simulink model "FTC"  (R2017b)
settings: Solver=FixedStepDiscrete  StartTime=0.0  StopTime=10.0  FixedStep=0.01  RelTol=1e-3  EnableMultiTasking=on
undefined symbols (not defined in the file): ASWTYPE_TRUE, Enum_CMSHVBatFltSevrtyStat
libraries: AIWAYS_Powertrain_BMS_lib x22

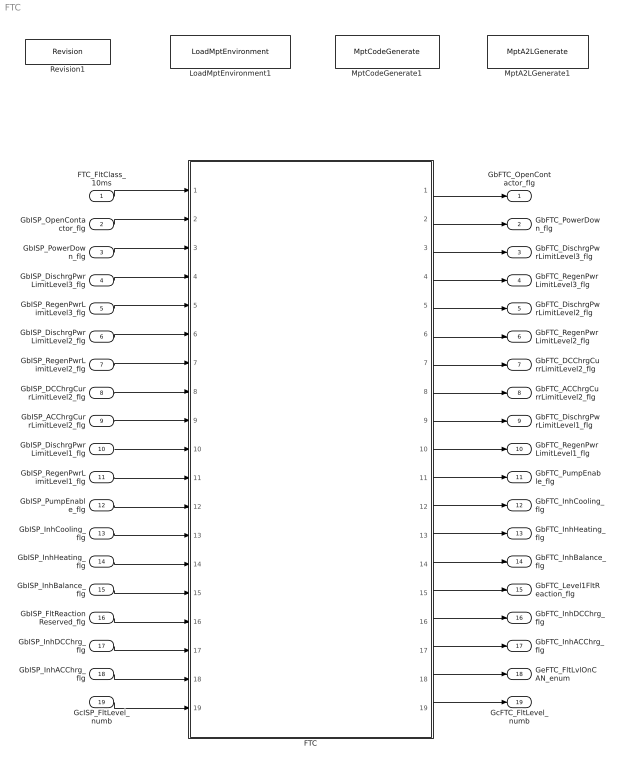
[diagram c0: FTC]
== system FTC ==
  FTC_FltClass_10ms : Inport
  GbISP_OpenContactor_flg : Inport  Port=2
  GbISP_PowerDown_flg : Inport  Port=3
  GbISP_DischrgPwrLimitLevel3_flg : Inport  Port=4
  GbISP_RegenPwrLimitLevel3_flg : Inport  Port=5
  GbISP_DischrgPwrLimitLevel2_flg : Inport  Port=6
  GbISP_RegenPwrLimitLevel2_flg : Inport  Port=7
  GbISP_DCChrgCurrLimitLevel2_flg : Inport  Port=8
  GbISP_ACChrgCurrLimitLevel2_flg : Inport  Port=9
  GbISP_DischrgPwrLimitLevel1_flg : Inport  Port=10
  GbISP_RegenPwrLimitLevel1_flg : Inport  Port=11
  GbISP_PumpEnable_flg : Inport  Port=12
  GbISP_InhCooling_flg : Inport  Port=13
  GbISP_InhHeating_flg : Inport  Port=14
  GbISP_InhBalance_flg : Inport  Port=15
  GbISP_FltReactionReserved_flg : Inport  Port=16
  GbISP_InhDCChrg_flg : Inport  Port=17
  GbISP_InhACChrg_flg : Inport  Port=18
  GcISP_FltLevel_numb : Inport  Port=19
  FTC : Subsystem
  LoadMptEnvironment1 : AIWAYS_Powertrain_BMS_lib/Config/LoadMptEnvironment  ProjectName=Comm  SuppierID=NewPlatformUAES
  MptA2LGenerate1 : AIWAYS_Powertrain_BMS_lib/Config/MptA2LGenerate  SystemSampleTime=-1
  MptCodeGenerate1 : AIWAYS_Powertrain_BMS_lib/Config/MptCodeGenerate  SystemSampleTime=-1
  Revision1 : AIWAYS_Powertrain_BMS_lib/Config/Revision  curVersion='M103C105'  newVersion='M103C105'
  GbFTC_OpenContactor_flg : Outport
  GbFTC_PowerDown_flg : Outport  Port=2
  GbFTC_DischrgPwrLimitLevel3_flg : Outport  Port=3
  GbFTC_RegenPwrLimitLevel3_flg : Outport  Port=4
  GbFTC_DischrgPwrLimitLevel2_flg : Outport  Port=5
  GbFTC_RegenPwrLimitLevel2_flg : Outport  Port=6
  GbFTC_DCChrgCurrLimitLevel2_flg : Outport  Port=7
  GbFTC_ACChrgCurrLimitLevel2_flg : Outport  Port=8
  GbFTC_DischrgPwrLimitLevel1_flg : Outport  Port=9
  GbFTC_RegenPwrLimitLevel1_flg : Outport  Port=10
  GbFTC_PumpEnable_flg : Outport  Port=11
  GbFTC_InhCooling_flg : Outport  Port=12
  GbFTC_InhHeating_flg : Outport  Port=13
  GbFTC_InhBalance_flg : Outport  Port=14
  GbFTC_Level1FltReaction_flg : Outport  Port=15
  GbFTC_InhDCChrg_flg : Outport  Port=16
  GbFTC_InhACChrg_flg : Outport  Port=17
  GeFTC_FltLvlOnCAN_enum : Outport  Port=18
  GcFTC_FltLevel_numb : Outport  Port=19
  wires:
  FTC_FltClass_10ms/1 -> FTC/1(FTC_FltClass_10ms)
  GbISP_OpenContactor_flg/1 -> FTC/2(GbISP_OpenContactor_flg)
  GbISP_PowerDown_flg/1 -> FTC/3(GbISP_PowerDown_flg)
  GbISP_DischrgPwrLimitLevel3_flg/1 -> FTC/4(GbISP_DischrgPwrLimitLevel3_flg)
  GbISP_RegenPwrLimitLevel3_flg/1 -> FTC/5(GbISP_RegenPwrLimitLevel3_flg)
  GbISP_DischrgPwrLimitLevel2_flg/1 -> FTC/6(GbISP_DischrgPwrLimitLevel2_flg)
  GbISP_RegenPwrLimitLevel2_flg/1 -> FTC/7(GbISP_RegenPwrLimitLevel2_flg)
  GbISP_DCChrgCurrLimitLevel2_flg/1 -> FTC/8(GbISP_DCChrgCurrLimitLevel2_flg)
  GbISP_ACChrgCurrLimitLevel2_flg/1 -> FTC/9(GbISP_ACChrgCurrLimitLevel2_flg)
  GbISP_DischrgPwrLimitLevel1_flg/1 -> FTC/10(GbISP_DischrgPwrLimitLevel1_flg)
  GbISP_RegenPwrLimitLevel1_flg/1 -> FTC/11(GbISP_RegenPwrLimitLevel1_flg)
  GbISP_PumpEnable_flg/1 -> FTC/12(GbISP_PumpEnable_flg)
  GbISP_InhCooling_flg/1 -> FTC/13(GbISP_InhCooling_flg)
  GbISP_InhHeating_flg/1 -> FTC/14(GbISP_InhHeating_flg)
  GbISP_InhBalance_flg/1 -> FTC/15(GbISP_InhBalance_flg)
  GbISP_FltReactionReserved_flg/1 -> FTC/16(GbISP_Level1FltReaction_flg)
  FTC/1(GbFTC_OpenContactor_flg) -> GbFTC_OpenContactor_flg/1
  FTC/2(GbFTC_PowerDown_flg) -> GbFTC_PowerDown_flg/1
  FTC/3(GbFTC_DischrgPwrLimitLevel3_flg) -> GbFTC_DischrgPwrLimitLevel3_flg/1
  FTC/4(GbFTC_RegenPwrLimitLevel3_flg) -> GbFTC_RegenPwrLimitLevel3_flg/1
  FTC/5(GbFTC_DischrgPwrLimitLevel2_flg) -> GbFTC_DischrgPwrLimitLevel2_flg/1
  FTC/6(GbFTC_RegenPwrLimitLevel2_flg) -> GbFTC_RegenPwrLimitLevel2_flg/1
  FTC/7(GbFTC_DCChrgCurrLimitLevel2_flg) -> GbFTC_DCChrgCurrLimitLevel2_flg/1
  FTC/8(GbFTC_ACChrgCurrLimitLevel2_flg) -> GbFTC_ACChrgCurrLimitLevel2_flg/1
  FTC/9(GbFTC_DischrgPwrLimitLevel1_flg) -> GbFTC_DischrgPwrLimitLevel1_flg/1
  FTC/10(GbFTC_RegenPwrLimitLevel1_flg) -> GbFTC_RegenPwrLimitLevel1_flg/1
  FTC/11(GbFTC_PumpEnable_flg) -> GbFTC_PumpEnable_flg/1
  FTC/12(GbFTC_InhCooling_flg) -> GbFTC_InhCooling_flg/1
  FTC/13(GbFTC_InhHeating_flg) -> GbFTC_InhHeating_flg/1
  FTC/14(GbFTC_InhBalance_flg) -> GbFTC_InhBalance_flg/1
  FTC/15(GbFTC_Level1FltReaction_flg) -> GbFTC_Level1FltReaction_flg/1
  FTC/16(GbFTC_InhDCChrg_flg) -> GbFTC_InhDCChrg_flg/1
  FTC/17(GbFTC_InhACChrg_flg) -> GbFTC_InhACChrg_flg/1
  GbISP_InhDCChrg_flg/1 -> FTC/17(GbISP_InhDCChrg_flg)
  GbISP_InhACChrg_flg/1 -> FTC/18(GbISP_InhACChrg_flg)
  FTC/18(GeFTC_FltLvlOnCAN_enum) -> GeFTC_FltLvlOnCAN_enum/1
  GcISP_FltLevel_numb/1 -> FTC/19(GcISP_FltLevel_numb)
  FTC/19(GcFTC_FltLevel_numb) -> GcFTC_FltLevel_numb/1

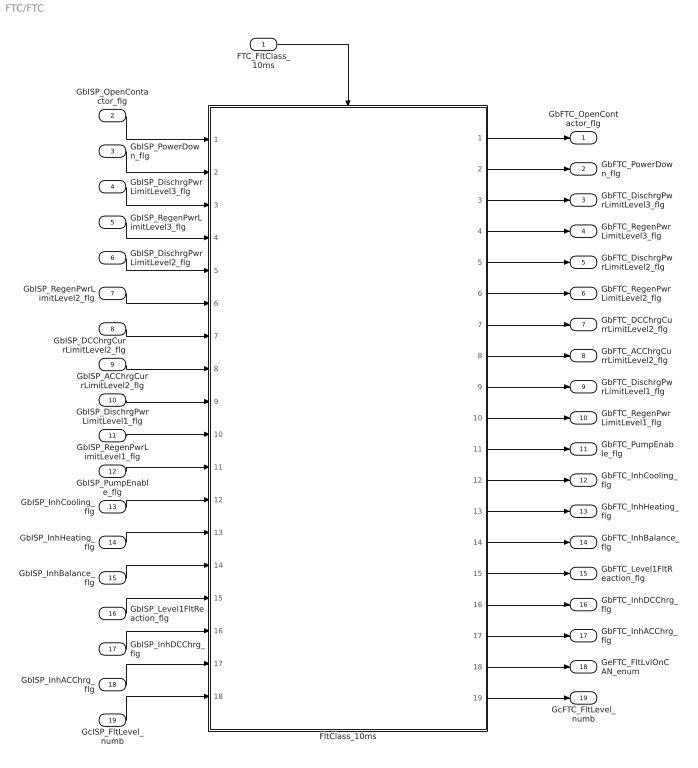
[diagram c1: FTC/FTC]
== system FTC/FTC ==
  FTC_FltClass_10ms : Inport
  GbISP_OpenContactor_flg : Inport  Port=2
  GbISP_PowerDown_flg : Inport  Port=3
  GbISP_DischrgPwrLimitLevel3_flg : Inport  Port=4
  GbISP_RegenPwrLimitLevel3_flg : Inport  Port=5
  GbISP_DischrgPwrLimitLevel2_flg : Inport  Port=6
  GbISP_RegenPwrLimitLevel2_flg : Inport  Port=7
  GbISP_DCChrgCurrLimitLevel2_flg : Inport  Port=8
  GbISP_ACChrgCurrLimitLevel2_flg : Inport  Port=9
  GbISP_DischrgPwrLimitLevel1_flg : Inport  Port=10
  GbISP_RegenPwrLimitLevel1_flg : Inport  Port=11
  GbISP_PumpEnable_flg : Inport  Port=12
  GbISP_InhCooling_flg : Inport  Port=13
  GbISP_InhHeating_flg : Inport  Port=14
  GbISP_InhBalance_flg : Inport  Port=15
  GbISP_Level1FltReaction_flg : Inport  Port=16
  GbISP_InhDCChrg_flg : Inport  Port=17
  GbISP_InhACChrg_flg : Inport  Port=18
  GcISP_FltLevel_numb : Inport  Port=19
  FltClass_10ms : Subsystem
  GbFTC_OpenContactor_flg : Outport
  GbFTC_PowerDown_flg : Outport  Port=2
  GbFTC_DischrgPwrLimitLevel3_flg : Outport  Port=3
  GbFTC_RegenPwrLimitLevel3_flg : Outport  Port=4
  GbFTC_DischrgPwrLimitLevel2_flg : Outport  Port=5
  GbFTC_RegenPwrLimitLevel2_flg : Outport  Port=6
  GbFTC_DCChrgCurrLimitLevel2_flg : Outport  Port=7
  GbFTC_ACChrgCurrLimitLevel2_flg : Outport  Port=8
  GbFTC_DischrgPwrLimitLevel1_flg : Outport  Port=9
  GbFTC_RegenPwrLimitLevel1_flg : Outport  Port=10
  GbFTC_PumpEnable_flg : Outport  Port=11
  GbFTC_InhCooling_flg : Outport  Port=12
  GbFTC_InhHeating_flg : Outport  Port=13
  GbFTC_InhBalance_flg : Outport  Port=14
  GbFTC_Level1FltReaction_flg : Outport  Port=15
  GbFTC_InhDCChrg_flg : Outport  Port=16
  GbFTC_InhACChrg_flg : Outport  Port=17
  GeFTC_FltLvlOnCAN_enum : Outport  Port=18
  GcFTC_FltLevel_numb : Outport  Port=19
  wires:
  GbISP_OpenContactor_flg/1 -> FltClass_10ms/1(GbISP_OpenContactor_flg)
  GbISP_PowerDown_flg/1 -> FltClass_10ms/2(GbISP_PowerDown_flg)
  GbISP_DischrgPwrLimitLevel3_flg/1 -> FltClass_10ms/3(GbISP_DischrgPwrLimitLevel3_flg)
  GbISP_RegenPwrLimitLevel3_flg/1 -> FltClass_10ms/4(GbISP_RegenPwrLimitLevel3_flg)
  GbISP_DischrgPwrLimitLevel2_flg/1 -> FltClass_10ms/5(GbISP_DischrgPwrLimitLevel2_flg)
  GbISP_RegenPwrLimitLevel2_flg/1 -> FltClass_10ms/6(GbISP_RegenPwrLimitLevel2_flg)
  GbISP_DCChrgCurrLimitLevel2_flg/1 -> FltClass_10ms/7(GbISP_DCChrgCurrLimitLevel2_flg)
  GbISP_ACChrgCurrLimitLevel2_flg/1 -> FltClass_10ms/8(GbISP_ACChrgCurrLimitLevel2_flg)
  GbISP_DischrgPwrLimitLevel1_flg/1 -> FltClass_10ms/9(GbISP_DischrgPwrLimitLevel1_flg)
  GbISP_RegenPwrLimitLevel1_flg/1 -> FltClass_10ms/10(GbISP_RegenPwrLimitLevel1_flg)
  GbISP_PumpEnable_flg/1 -> FltClass_10ms/11(GbISP_PumpEnable_flg)
  GbISP_InhCooling_flg/1 -> FltClass_10ms/12(GbISP_InhCooling_flg)
  GbISP_InhHeating_flg/1 -> FltClass_10ms/13(GbISP_InhHeating_flg)
  GbISP_InhBalance_flg/1 -> FltClass_10ms/14(GbISP_InhBalance_flg)
  GbISP_Level1FltReaction_flg/1 -> FltClass_10ms/15(GbISP_Level1FltReaction_flg)
  FltClass_10ms/1(GbFTC_OpenContactor_flg) -> GbFTC_OpenContactor_flg/1
  FltClass_10ms/2(GbFTC_PowerDown_flg) -> GbFTC_PowerDown_flg/1
  FltClass_10ms/3(GbFTC_DischrgPwrLimitLevel3_flg) -> GbFTC_DischrgPwrLimitLevel3_flg/1
  FltClass_10ms/4(GbFTC_RegenPwrLimitLevel3_flg) -> GbFTC_RegenPwrLimitLevel3_flg/1
  FltClass_10ms/5(GbFTC_DischrgPwrLimitLevel2_flg) -> GbFTC_DischrgPwrLimitLevel2_flg/1
  FltClass_10ms/6(GbFTC_RegenPwrLimitLevel2_flg) -> GbFTC_RegenPwrLimitLevel2_flg/1
  FltClass_10ms/7(GbFTC_DCChrgCurrLimitLevel2_flg) -> GbFTC_DCChrgCurrLimitLevel2_flg/1
  FltClass_10ms/8(GbFTC_ACChrgCurrLimitLevel2_flg) -> GbFTC_ACChrgCurrLimitLevel2_flg/1
  FltClass_10ms/9(GbFTC_DischrgPwrLimitLevel1_flg) -> GbFTC_DischrgPwrLimitLevel1_flg/1
  FltClass_10ms/10(GbFTC_RegenPwrLimitLevel1_flg) -> GbFTC_RegenPwrLimitLevel1_flg/1
  FltClass_10ms/11(GbFTC_PumpEnable_flg) -> GbFTC_PumpEnable_flg/1
  FltClass_10ms/12(GbFTC_InhCooling_flg) -> GbFTC_InhCooling_flg/1
  FltClass_10ms/13(GbFTC_InhHeating_flg) -> GbFTC_InhHeating_flg/1
  FltClass_10ms/14(GbFTC_InhBalance_flg) -> GbFTC_InhBalance_flg/1
  FltClass_10ms/15(GbFTC_Level1FltReaction_flg) -> GbFTC_Level1FltReaction_flg/1
  FTC_FltClass_10ms/1 -> FltClass_10ms/Trigger
  GbISP_InhDCChrg_flg/1 -> FltClass_10ms/16(GbISP_InhDCChrg_flg)
  GbISP_InhACChrg_flg/1 -> FltClass_10ms/17(GbISP_InhACChrg_flg)
  FltClass_10ms/16(GbFTC_InhDCChrg_flg) -> GbFTC_InhDCChrg_flg/1
  FltClass_10ms/17(GbFTC_InhACChrg_flg) -> GbFTC_InhACChrg_flg/1
  FltClass_10ms/18(GeFTC_FltLvlOnCAN_enum) -> GeFTC_FltLvlOnCAN_enum/1
  GcISP_FltLevel_numb/1 -> FltClass_10ms/18(GcISP_FltLevel_numb)
  FltClass_10ms/19(GcFTC_FltLevel_numb) -> GcFTC_FltLevel_numb/1

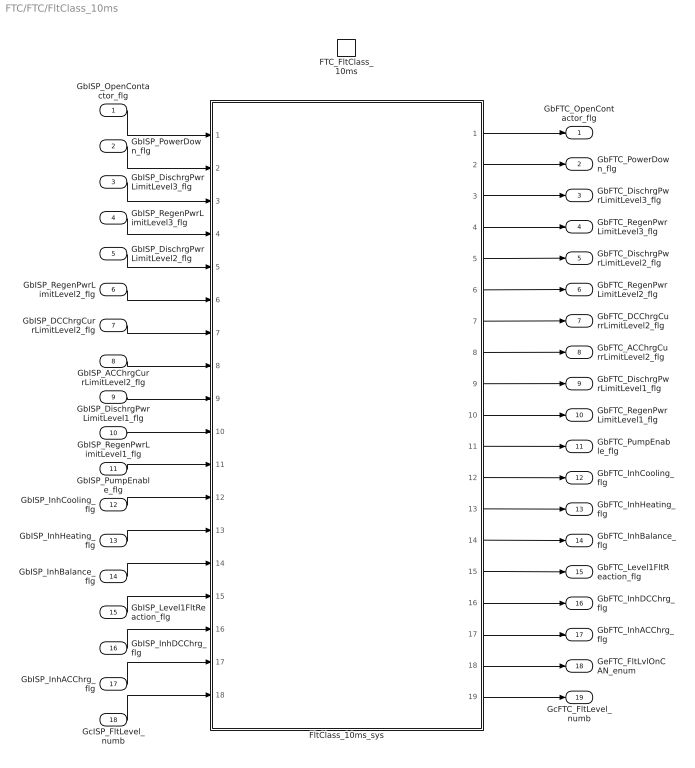
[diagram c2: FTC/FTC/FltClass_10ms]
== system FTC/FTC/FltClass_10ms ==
  GbISP_OpenContactor_flg : Inport
  GbISP_PowerDown_flg : Inport  Port=2
  GbISP_DischrgPwrLimitLevel3_flg : Inport  Port=3
  GbISP_RegenPwrLimitLevel3_flg : Inport  Port=4
  GbISP_DischrgPwrLimitLevel2_flg : Inport  Port=5
  GbISP_RegenPwrLimitLevel2_flg : Inport  Port=6
  GbISP_DCChrgCurrLimitLevel2_flg : Inport  Port=7
  GbISP_ACChrgCurrLimitLevel2_flg : Inport  Port=8
  GbISP_DischrgPwrLimitLevel1_flg : Inport  Port=9
  GbISP_RegenPwrLimitLevel1_flg : Inport  Port=10
  GbISP_PumpEnable_flg : Inport  Port=11
  GbISP_InhCooling_flg : Inport  Port=12
  GbISP_InhHeating_flg : Inport  Port=13
  GbISP_InhBalance_flg : Inport  Port=14
  GbISP_Level1FltReaction_flg : Inport  Port=15
  GbISP_InhDCChrg_flg : Inport  Port=16
  GbISP_InhACChrg_flg : Inport  Port=17
  GcISP_FltLevel_numb : Inport  Port=18
  FTC_FltClass_10ms : TriggerPort  TriggerType=function-call  VariantControl=(inherit)
  FltClass_10ms_sys : Subsystem
  GbFTC_OpenContactor_flg : Outport
  GbFTC_PowerDown_flg : Outport  Port=2
  GbFTC_DischrgPwrLimitLevel3_flg : Outport  Port=3
  GbFTC_RegenPwrLimitLevel3_flg : Outport  Port=4
  GbFTC_DischrgPwrLimitLevel2_flg : Outport  Port=5
  GbFTC_RegenPwrLimitLevel2_flg : Outport  Port=6
  GbFTC_DCChrgCurrLimitLevel2_flg : Outport  Port=7
  GbFTC_ACChrgCurrLimitLevel2_flg : Outport  Port=8
  GbFTC_DischrgPwrLimitLevel1_flg : Outport  Port=9
  GbFTC_RegenPwrLimitLevel1_flg : Outport  Port=10
  GbFTC_PumpEnable_flg : Outport  Port=11
  GbFTC_InhCooling_flg : Outport  Port=12
  GbFTC_InhHeating_flg : Outport  Port=13
  GbFTC_InhBalance_flg : Outport  Port=14
  GbFTC_Level1FltReaction_flg : Outport  Port=15
  GbFTC_InhDCChrg_flg : Outport  Port=16
  GbFTC_InhACChrg_flg : Outport  Port=17
  GeFTC_FltLvlOnCAN_enum : Outport  Port=18
  GcFTC_FltLevel_numb : Outport  Port=19
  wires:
  FltClass_10ms_sys/1(GbFTC_OpenContactor_flg) -> GbFTC_OpenContactor_flg/1
  FltClass_10ms_sys/2(GbFTC_PowerDown_flg) -> GbFTC_PowerDown_flg/1
  FltClass_10ms_sys/3(GbFTC_DischrgPwrLimitLevel3_flg) -> GbFTC_DischrgPwrLimitLevel3_flg/1
  FltClass_10ms_sys/4(GbFTC_RegenPwrLimitLevel3_flg) -> GbFTC_RegenPwrLimitLevel3_flg/1
  FltClass_10ms_sys/5(GbFTC_DischrgPwrLimitLevel2_flg) -> GbFTC_DischrgPwrLimitLevel2_flg/1
  FltClass_10ms_sys/6(GbFTC_RegenPwrLimitLevel2_flg) -> GbFTC_RegenPwrLimitLevel2_flg/1
  FltClass_10ms_sys/7(GbFTC_DCChrgCurrLimitLevel2_flg) -> GbFTC_DCChrgCurrLimitLevel2_flg/1
  FltClass_10ms_sys/8(GbFTC_ACChrgCurrLimitLevel2_flg) -> GbFTC_ACChrgCurrLimitLevel2_flg/1
  FltClass_10ms_sys/9(GbFTC_DischrgPwrLimitLevel1_flg) -> GbFTC_DischrgPwrLimitLevel1_flg/1
  FltClass_10ms_sys/10(GbFTC_RegenPwrLimitLevel1_flg) -> GbFTC_RegenPwrLimitLevel1_flg/1
  FltClass_10ms_sys/11(GbFTC_PumpEnable_flg) -> GbFTC_PumpEnable_flg/1
  FltClass_10ms_sys/12(GbFTC_InhCooling_flg) -> GbFTC_InhCooling_flg/1
  FltClass_10ms_sys/13(GbFTC_InhHeating_flg) -> GbFTC_InhHeating_flg/1
  FltClass_10ms_sys/14(GbFTC_InhBalance_flg) -> GbFTC_InhBalance_flg/1
  FltClass_10ms_sys/15(GbFTC_Level1FltReaction_flg) -> GbFTC_Level1FltReaction_flg/1
  GbISP_PowerDown_flg/1 -> FltClass_10ms_sys/2(GbISP_PowerDown_flg)
  GbISP_OpenContactor_flg/1 -> FltClass_10ms_sys/1(GbISP_OpenContactor_flg)
  GbISP_DischrgPwrLimitLevel3_flg/1 -> FltClass_10ms_sys/3(GbISP_DischrgPwrLimitLevel3_flg)
  GbISP_RegenPwrLimitLevel3_flg/1 -> FltClass_10ms_sys/4(GbISP_RegenPwrLimitLevel3_flg)
  GbISP_DischrgPwrLimitLevel2_flg/1 -> FltClass_10ms_sys/5(GbISP_DischrgPwrLimitLevel2_flg)
  GbISP_RegenPwrLimitLevel2_flg/1 -> FltClass_10ms_sys/6(GbISP_RegenPwrLimitLevel2_flg)
  GbISP_DCChrgCurrLimitLevel2_flg/1 -> FltClass_10ms_sys/7(GbISP_DCChrgCurrLimitLevel2_flg)
  GbISP_ACChrgCurrLimitLevel2_flg/1 -> FltClass_10ms_sys/8(GbISP_ACChrgCurrLimitLevel2_flg)
  GbISP_DischrgPwrLimitLevel1_flg/1 -> FltClass_10ms_sys/9(GbISP_DischrgPwrLimitLevel1_flg)
  GbISP_RegenPwrLimitLevel1_flg/1 -> FltClass_10ms_sys/10(GbISP_RegenPwrLimitLevel1_flg)
  GbISP_PumpEnable_flg/1 -> FltClass_10ms_sys/11(GbISP_PumpEnable_flg)
  GbISP_InhCooling_flg/1 -> FltClass_10ms_sys/12(GbISP_InhCooling_flg)
  GbISP_InhHeating_flg/1 -> FltClass_10ms_sys/13(GbISP_InhHeating_flg)
  GbISP_InhBalance_flg/1 -> FltClass_10ms_sys/14(GbISP_InhBalance_flg)
  GbISP_Level1FltReaction_flg/1 -> FltClass_10ms_sys/15(GbISP_Level1FltReaction_flg)
  GbISP_InhDCChrg_flg/1 -> FltClass_10ms_sys/16(GbISP_InhDCChrg_flg)
  GbISP_InhACChrg_flg/1 -> FltClass_10ms_sys/17(GbISP_InhACChrg_flg)
  FltClass_10ms_sys/16(GbFTC_InhDCChrg_flg) -> GbFTC_InhDCChrg_flg/1
  FltClass_10ms_sys/17(GbFTC_InhACChrg_flg) -> GbFTC_InhACChrg_flg/1
  FltClass_10ms_sys/18(GeFTC_FltLvlOnCAN_enum) -> GeFTC_FltLvlOnCAN_enum/1
  GcISP_FltLevel_numb/1 -> FltClass_10ms_sys/18(GcISP_FltLevel_numb)
  FltClass_10ms_sys/19(GcFTC_FltLevel_numb) -> GcFTC_FltLevel_numb/1

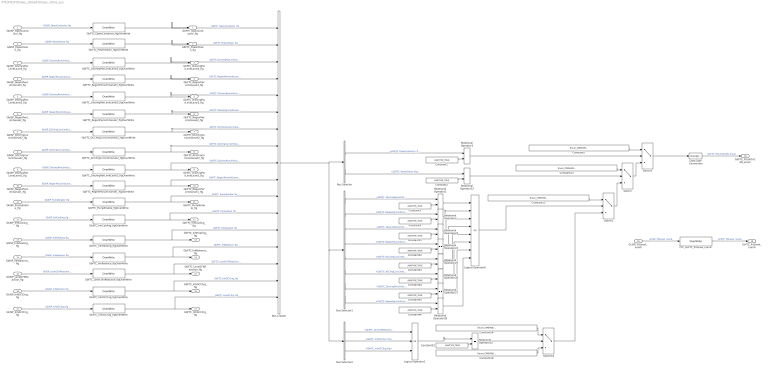
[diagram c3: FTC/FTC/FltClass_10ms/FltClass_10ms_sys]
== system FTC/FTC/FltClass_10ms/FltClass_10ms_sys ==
  GbISP_OpenContactor_flg : Inport
  GbISP_PowerDown_flg : Inport  Port=2
  GbISP_DischrgPwrLimitLevel3_flg : Inport  Port=3
  GbISP_RegenPwrLimitLevel3_flg : Inport  Port=4
  GbISP_DischrgPwrLimitLevel2_flg : Inport  Port=5
  GbISP_RegenPwrLimitLevel2_flg : Inport  Port=6
  GbISP_DCChrgCurrLimitLevel2_flg : Inport  Port=7
  GbISP_ACChrgCurrLimitLevel2_flg : Inport  Port=8
  GbISP_DischrgPwrLimitLevel1_flg : Inport  Port=9
  GbISP_RegenPwrLimitLevel1_flg : Inport  Port=10
  GbISP_PumpEnable_flg : Inport  Port=11
  GbISP_InhCooling_flg : Inport  Port=12
  GbISP_InhHeating_flg : Inport  Port=13
  GbISP_InhBalance_flg : Inport  Port=14
  GbISP_Level1FltReaction_flg : Inport  Port=15
  GbISP_InhDCChrg_flg : Inport  Port=16
  GbISP_InhACChrg_flg : Inport  Port=17
  GcISP_FltLevel_numb : Inport  Port=18
  Bus Creator : BusCreator  Inputs=17
  Bus Selector : BusSelector  OutputSignals=GbFTC_OpenContactor_flg,GbFTC_PowerDown_flg
  Bus Selector1 : BusSelector  OutputSignals=GbFTC_DischrgPwrLimitLevel3_flg,GbFTC_RegenPwrLimitLevel3_flg,GbFTC_DischrgPwrLimitLevel2_flg,GbFTC_RegenPwrLimitLevel2_flg,GbFTC_DCChrgCurrLimitLevel2_flg,GbFTC_ACChrgCurrLimitLevel2_flg,GbFTC_DischrgPwrLimitLevel1_flg,GbFTC_RegenPwrLimitLevel1_flg
  Bus Selector2 : BusSelector  OutputSignals=GbFTC_Level1FltReaction_flg,GbFTC_InhDCChrg_flg,GbFTC_InhACChrg_flg
  Constant{1..4,11,42..46,52} (11 alike) : Constant  Value=ASWTYPE_TRUE
  Constant10 : Constant  Value=Enum_CMSHVBatFltSevrtyStat.Enum_CMSHVBatFltSevrtyStat_Default
  Constant12 : Constant  Value=Enum_CMSHVBatFltSevrtyStat.Enum_CMSHVBatFltSevrtyStat_Med
  Constant13 : Constant  Value=Enum_CMSHVBatFltSevrtyStat.Enum_CMSHVBatFltSevrtyStat_High
  Constant5 : Constant  Value=Enum_CMSHVBatFltSevrtyStat.Enum_CMSHVBatFltSevrtyStat_Highest
  Constant56 : Constant  Value=Enum_CMSHVBatFltSevrtyStat.Enum_CMSHVBatFltSevrtyStat_Low
  Data Type Conversion : DataTypeConversion
  FTC_GcFTC_FltLevel_numb : AIWAYS_Powertrain_BMS_lib/Signals/OverWrite  OverWrite_Value=CcFTC_FltLevelOvr_numb  OverWrite_flag=CbFTC_FltLevelOvrSwt_flg
  GbFTC_ACChrgCurrLimitLevel2_flgOverWrite : AIWAYS_Powertrain_BMS_lib/Signals/OverWrite  OverWrite_Value=CbFTC_ACChrgCurrLimitLevel2Ovr_flg  OverWrite_flag=CbFTC_ACChrgCurrLimitLevel2OvrSwt_flg
  GbFTC_DCChrgCurrLimitLevel2_flgOverWrite : AIWAYS_Powertrain_BMS_lib/Signals/OverWrite  OverWrite_Value=CbFTC_DCChrgCurrLimitLevel2Ovr_flg  OverWrite_flag=CbFTC_DCChrgCurrLimitLevel2OvrSwt_flg
  GbFTC_DischrgPwrLimitLevel1_flgOverWrite : AIWAYS_Powertrain_BMS_lib/Signals/OverWrite  OverWrite_Value=CbFTC_DischrgPwrLimitLevel1Ovr_flg  OverWrite_flag=CbFTC_DischrgPwrLimitLevel1OvrSwt_flg
  GbFTC_DischrgPwrLimitLevel2_flgOverWrite : AIWAYS_Powertrain_BMS_lib/Signals/OverWrite  OverWrite_Value=CbFTC_DischrgPwrLimitLevel2Ovr_flg  OverWrite_flag=CbFTC_DischrgPwrLimitLevel2OvrSwt_flg
  GbFTC_DischrgPwrLimitLevel3_flgOverWrite : AIWAYS_Powertrain_BMS_lib/Signals/OverWrite  OverWrite_Value=CbFTC_DischrgPwrLimitLevel3Ovr_flg  OverWrite_flag=CbFTC_DischrgPwrLimitLevel3OvrSwt_flg
  GbFTC_InhACChrg_flgOverWrite : AIWAYS_Powertrain_BMS_lib/Signals/OverWrite  OverWrite_Value=CbFTC_InhACChrgOvr_flg  OverWrite_flag=CbFTC_InhACChrgOvrSwt_flg
  GbFTC_InhBalance_flgOverWrite : AIWAYS_Powertrain_BMS_lib/Signals/OverWrite  OverWrite_Value=CbFTC_InhBalanceOvr_flg  OverWrite_flag=CbFTC_InhBalanceOvrSwt_flg
  GbFTC_InhCooling_flgOverWrite : AIWAYS_Powertrain_BMS_lib/Signals/OverWrite  OverWrite_Value=CbFTC_InhCoolingOvr_flg  OverWrite_flag=CbFTC_InhCoolingOvrSwt_flg
  GbFTC_InhDCChrg_flgOverWrite : AIWAYS_Powertrain_BMS_lib/Signals/OverWrite  OverWrite_Value=CbFTC_InhDCChrgOvr_flg  OverWrite_flag=CbFTC_InhDCChrgOvrSwt_flg
  GbFTC_InhHeating_flgOverWrite : AIWAYS_Powertrain_BMS_lib/Signals/OverWrite  OverWrite_Value=CbFTC_InhHeatingOvr_flg  OverWrite_flag=CbFTC_InhHeatingOvrSwt_flg
  GbFTC_Level1FltReaction_flgOverWrite : AIWAYS_Powertrain_BMS_lib/Signals/OverWrite  OverWrite_Value=CbFTC_Level1FltReactionOvr_flg  OverWrite_flag=CbFTC_Level1FltReactionOvrSwt_flg
  GbFTC_OpenContactor_flgOverWrite : AIWAYS_Powertrain_BMS_lib/Signals/OverWrite  OverWrite_Value=CbFTC_OpenContactorOvr_flg  OverWrite_flag=CbFTC_OpenContactorOvrSwt_flg
  GbFTC_PowerDown_flgOverWrite : AIWAYS_Powertrain_BMS_lib/Signals/OverWrite  OverWrite_Value=CbFTC_PowerDownOvr_flg  OverWrite_flag=CbFTC_PowerDownOvrSwt_flg
  GbFTC_PumpEnable_flgOverWrite : AIWAYS_Powertrain_BMS_lib/Signals/OverWrite  OverWrite_Value=CbFTC_PumpEnableOvr_flg  OverWrite_flag=CbFTC_PumpEnableOvrSwt_flg
  GbFTC_RegenPwrLimitLevel1_flgOverWrite : AIWAYS_Powertrain_BMS_lib/Signals/OverWrite  OverWrite_Value=CbFTC_RegenPwrLimitLevel1Ovr_flg  OverWrite_flag=CbFTC_RegenPwrLimitLevel1OvrSwt_flg
  GbFTC_RegenPwrLimitLevel2_flgOverWrite : AIWAYS_Powertrain_BMS_lib/Signals/OverWrite  OverWrite_Value=CbFTC_RegenPwrLimitLevel2Ovr_flg  OverWrite_flag=CbFTC_RegenPwrLimitLevel2OvrSwt_flg
  GbFTC_RegenPwrLimitLevel3_flgOverWrite : AIWAYS_Powertrain_BMS_lib/Signals/OverWrite  OverWrite_Value=CbFTC_RegenPwrLimitLevel3Ovr_flg  OverWrite_flag=CbFTC_RegenPwrLimitLevel3OvrSwt_flg
  Logical Operator1 : Logic  Operator=OR  Inputs=3  AllPortsSameDT=off  OutDataTypeStr=boolean
  Logical Operator6 : Logic  Operator=OR  Inputs=8  AllPortsSameDT=off  OutDataTypeStr=boolean
  Relational Operator{1..3,22..28,32} (11 alike) : RelationalOperator  Operator===  OutDataTypeStr=boolean
  Switch{,1,3,18} (4 alike) : Switch  Criteria=u2 ~= 0
  GbFTC_OpenContactor_flg : Outport
  GbFTC_PowerDown_flg : Outport  Port=2
  GbFTC_DischrgPwrLimitLevel3_flg : Outport  Port=3
  GbFTC_RegenPwrLimitLevel3_flg : Outport  Port=4
  GbFTC_DischrgPwrLimitLevel2_flg : Outport  Port=5
  GbFTC_RegenPwrLimitLevel2_flg : Outport  Port=6
  GbFTC_DCChrgCurrLimitLevel2_flg : Outport  Port=7
  GbFTC_ACChrgCurrLimitLevel2_flg : Outport  Port=8
  GbFTC_DischrgPwrLimitLevel1_flg : Outport  Port=9
  GbFTC_RegenPwrLimitLevel1_flg : Outport  Port=10
  GbFTC_PumpEnable_flg : Outport  Port=11
  GbFTC_InhCooling_flg : Outport  Port=12
  GbFTC_InhHeating_flg : Outport  Port=13
  GbFTC_InhBalance_flg : Outport  Port=14
  GbFTC_Level1FltReaction_flg : Outport  Port=15
  GbFTC_InhDCChrg_flg : Outport  Port=16
  GbFTC_InhACChrg_flg : Outport  Port=17
  GeFTC_FltLvlOnCAN_enum : Outport  Port=18
  GcFTC_FltLevel_numb : Outport  Port=19
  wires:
  GbISP_OpenContactor_flg/1 -> GbFTC_OpenContactor_flgOverWrite/1  "GbISP_OpenContactor_flg"
  GbISP_PowerDown_flg/1 -> GbFTC_PowerDown_flgOverWrite/1  "GbISP_PowerDown_flg"
  GbISP_DischrgPwrLimitLevel3_flg/1 -> GbFTC_DischrgPwrLimitLevel3_flgOverWrite/1  "GbISP_DischrgPwrLimitLevel3_flg"
  GbFTC_DischrgPwrLimitLevel3_flgOverWrite/1 -> Bus Creator/3, GbFTC_DischrgPwrLimitLevel3_flg/1  "GbFTC_DischrgPwrLimitLevel3_flg"
  GbISP_RegenPwrLimitLevel3_flg/1 -> GbFTC_RegenPwrLimitLevel3_flgOverWrite/1  "GbISP_RegenPwrLimitLevel3_flg"
  GbFTC_RegenPwrLimitLevel3_flgOverWrite/1 -> Bus Creator/4, GbFTC_RegenPwrLimitLevel3_flg/1  "GbFTC_RegenPwrLimitLevel3_flg"
  GbISP_DischrgPwrLimitLevel2_flg/1 -> GbFTC_DischrgPwrLimitLevel2_flgOverWrite/1  "GbISP_DischrgPwrLimitLevel2_flg"
  GbFTC_DischrgPwrLimitLevel2_flgOverWrite/1 -> Bus Creator/5, GbFTC_DischrgPwrLimitLevel2_flg/1  "GbFTC_DischrgPwrLimitLevel2_flg"
  GbISP_RegenPwrLimitLevel2_flg/1 -> GbFTC_RegenPwrLimitLevel2_flgOverWrite/1  "GbISP_RegenPwrLimitLevel2_flg"
  GbFTC_RegenPwrLimitLevel2_flgOverWrite/1 -> GbFTC_RegenPwrLimitLevel2_flg/1, Bus Creator/6  "GbFTC_RegenPwrLimitLevel2_flg"
  GbISP_DCChrgCurrLimitLevel2_flg/1 -> GbFTC_DCChrgCurrLimitLevel2_flgOverWrite/1  "GbISP_DCChrgCurrLimitLevel2_flg"
  GbFTC_DCChrgCurrLimitLevel2_flgOverWrite/1 -> Bus Creator/7, GbFTC_DCChrgCurrLimitLevel2_flg/1  "GbFTC_DCChrgCurrLimitLevel2_flg"
  GbISP_ACChrgCurrLimitLevel2_flg/1 -> GbFTC_ACChrgCurrLimitLevel2_flgOverWrite/1  "GbISP_ACChrgCurrLimitLevel2_flg"
  GbISP_DischrgPwrLimitLevel1_flg/1 -> GbFTC_DischrgPwrLimitLevel1_flgOverWrite/1  "GbISP_DischrgPwrLimitLevel1_flg"
  GbISP_RegenPwrLimitLevel1_flg/1 -> GbFTC_RegenPwrLimitLevel1_flgOverWrite/1  "GbISP_RegenPwrLimitLevel1_flg"
  GbISP_PumpEnable_flg/1 -> GbFTC_PumpEnable_flgOverWrite/1  "GbISP_PumpEnable_flg"
  GbISP_InhCooling_flg/1 -> GbFTC_InhCooling_flgOverWrite/1  "GbISP_InhCooling_flg"
  GbISP_InhHeating_flg/1 -> GbFTC_InhHeating_flgOverWrite/1  "GbISP_InhHeating_flg"
  GbISP_InhBalance_flg/1 -> GbFTC_InhBalance_flgOverWrite/1  "GbISP_InhBalance_flg"
  GbISP_Level1FltReaction_flg/1 -> GbFTC_Level1FltReaction_flgOverWrite/1  "GbISP_Level1FltReaction_flg"
  GbFTC_ACChrgCurrLimitLevel2_flgOverWrite/1 -> GbFTC_ACChrgCurrLimitLevel2_flg/1, Bus Creator/8  "GbFTC_ACChrgCurrLimitLevel2_flg"
  GbFTC_DischrgPwrLimitLevel1_flgOverWrite/1 -> GbFTC_DischrgPwrLimitLevel1_flg/1, Bus Creator/9  "GbFTC_DischrgPwrLimitLevel1_flg"
  GbFTC_RegenPwrLimitLevel1_flgOverWrite/1 -> GbFTC_RegenPwrLimitLevel1_flg/1, Bus Creator/10  "GbFTC_RegenPwrLimitLevel1_flg"
  GbFTC_PumpEnable_flgOverWrite/1 -> GbFTC_PumpEnable_flg/1, Bus Creator/11  "GbFTC_PumpEnable_flg"
  GbFTC_InhCooling_flgOverWrite/1 -> Bus Creator/12, GbFTC_InhCooling_flg/1  "GbFTC_InhCooling_flg"
  GbFTC_InhHeating_flgOverWrite/1 -> Bus Creator/13, GbFTC_InhHeating_flg/1  "GbFTC_InhHeating_flg"
  GbFTC_InhBalance_flgOverWrite/1 -> Bus Creator/14, GbFTC_InhBalance_flg/1  "GbFTC_InhBalance_flg"
  GbFTC_Level1FltReaction_flgOverWrite/1 -> Bus Creator/15, GbFTC_Level1FltReaction_flg/1  "GbFTC_Level1FltReaction_flg"
  GbFTC_InhDCChrg_flgOverWrite/1 -> Bus Creator/16, GbFTC_InhDCChrg_flg/1  "GbFTC_InhDCChrg_flg"
  GbISP_InhDCChrg_flg/1 -> GbFTC_InhDCChrg_flgOverWrite/1  "GbISP_InhDCChrg_flg"
  GbISP_InhACChrg_flg/1 -> GbFTC_InhACChrg_flgOverWrite/1  "GbISP_InhACChrg_flg"
  GbFTC_InhACChrg_flgOverWrite/1 -> Bus Creator/17, GbFTC_InhACChrg_flg/1  "GbFTC_InhACChrg_flg"
  Relational Operator3/1 -> Switch3/2
  Constant43/1 -> Relational Operator25/2
  Constant5/1 -> Switch3/1
  Constant56/1 -> Switch18/1
  GbFTC_OpenContactor_flgOverWrite/1 -> Bus Creator/1, GbFTC_OpenContactor_flg/1  "GbFTC_OpenContactor_flg"
  GbFTC_PowerDown_flgOverWrite/1 -> Bus Creator/2, GbFTC_PowerDown_flg/1  "GbFTC_PowerDown_flg"
  Relational Operator32/1 -> Switch18/2
  Relational Operator27/1 -> Logical Operator6/7
  Constant42/1 -> Relational Operator24/2
  Logical Operator6/1 -> Switch1/2
  Logical Operator1/1 -> Relational Operator32/1
  Relational Operator1/1 -> Logical Operator6/1
  Constant52/1 -> Relational Operator32/2
  Switch18/1 -> Switch1/3
  Relational Operator26/1 -> Logical Operator6/6
  Constant46/1 -> Relational Operator28/2
  Relational Operator28/1 -> Logical Operator6/8
  Relational Operator23/1 -> Logical Operator6/3
  Relational Operator2/1 -> Logical Operator6/2
  Constant45/1 -> Relational Operator27/2
  Constant44/1 -> Relational Operator26/2
  Constant4/1 -> Relational Operator2/2
  Relational Operator25/1 -> Logical Operator6/5
  Constant12/1 -> Switch1/1
  Constant10/1 -> Switch18/3
  Constant11/1 -> Relational Operator23/2
  Relational Operator24/1 -> Logical Operator6/4
  Data Type Conversion/1 -> GeFTC_FltLvlOnCAN_enum/1  "GeFTC_FltLvlOnCAN_enum"
  Switch/1 -> Switch3/3
  Constant2/1 -> Relational Operator22/2
  Constant13/1 -> Switch/1
  Relational Operator22/1 -> Switch/2
  Constant3/1 -> Relational Operator1/2
  Constant1/1 -> Relational Operator3/2
  Switch1/1 -> Switch/3
  Bus Creator/1 -> Bus Selector2/1, Bus Selector1/1, Bus Selector/1
  Bus Selector/1 -> Relational Operator3/1  "<GbFTC_OpenContactor_flg>"
  Bus Selector/2 -> Relational Operator22/1  "<GbFTC_PowerDown_flg>"
  Bus Selector1/1 -> Relational Operator1/1  "<GbFTC_DischrgPwrLimitLevel3_flg>"
  Bus Selector1/2 -> Relational Operator2/1  "<GbFTC_RegenPwrLimitLevel3_flg>"
  Bus Selector1/3 -> Relational Operator23/1  "<GbFTC_DischrgPwrLimitLevel2_flg>"
  Bus Selector1/4 -> Relational Operator24/1  "<GbFTC_RegenPwrLimitLevel2_flg>"
  Bus Selector1/5 -> Relational Operator25/1  "<GbFTC_DCChrgCurrLimitLevel2_flg>"
  Bus Selector1/6 -> Relational Operator26/1  "<GbFTC_ACChrgCurrLimitLevel2_flg>"
  Bus Selector1/7 -> Relational Operator27/1  "<GbFTC_DischrgPwrLimitLevel1_flg>"
  Bus Selector1/8 -> Relational Operator28/1  "<GbFTC_RegenPwrLimitLevel1_flg>"
  Bus Selector2/1 -> Logical Operator1/1  "<GbFTC_Level1FltReaction_flg>"
  Bus Selector2/2 -> Logical Operator1/2  "<GbFTC_InhDCChrg_flg>"
  Bus Selector2/3 -> Logical Operator1/3  "<GbFTC_InhACChrg_flg>"
  Switch3/1 -> Data Type Conversion/1
  FTC_GcFTC_FltLevel_numb/1 -> GcFTC_FltLevel_numb/1  "GcFTC_FltLevel_numb"
  GcISP_FltLevel_numb/1 -> FTC_GcFTC_FltLevel_numb/1  "GcISP_FltLevel_numb"
